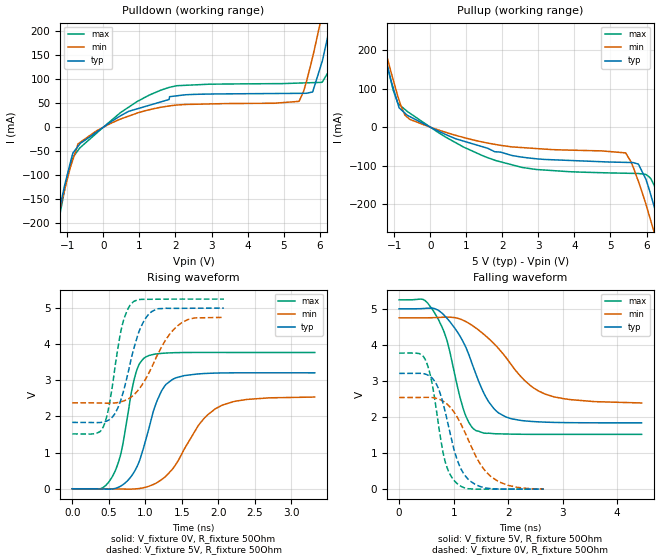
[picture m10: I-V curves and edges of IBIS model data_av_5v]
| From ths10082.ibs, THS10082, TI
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|   data_av_5v Model
[Model]   data_av_5v
Model_type   Output
Polarity   Non-Inverting
Vmeas = 2.5
Vref = 2.5
Cref = 2pF
Rref = 50
|   typ   min   max
C_comp   1.852e-12   1.852e-12   1.893e-12
[Voltage Range]   5   4.75   5.25
|Ambient Temperature   25   85   -40
|Junction Temperature
[Temperature Range]   27   125   -40
[Pullup Reference]   5   4.75   5.25
[Pulldown Reference]   0   0   0
[Power Clamp Reference]   5   4.75   5.25
[GND Clamp Reference]   0   0   0
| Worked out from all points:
|   slope of the pulldown table from 0 to 0.75 V, typ, clamps not added: 22.1 ohm
|   slope of the pullup table from 0 to 0.75 V, typ, clamps not added: 23.8 ohm
|   falling waveform, V_fixture 5V, R_fixture 50Ohm: 20-80 % time 559ps typ, 852ps min, 385ps max; typ from 5 V to 1.84 V
|   rising waveform, V_fixture 0V, R_fixture 50Ohm: 20-80 % time 298ps typ, 490ps min, 212ps max; typ from 0 V to 3.21 V
|   rising waveform, V_fixture 5V, R_fixture 50Ohm: 20-80 % time 251ps typ, 385ps min, 181ps max; typ from 1.84 V to 5 V
|   falling waveform, V_fixture 0V, R_fixture 50Ohm: 20-80 % time 339ps typ, 527ps min, 254ps max; typ from 3.21 V to 0 V
[Pulldown]
|   Voltage   I(typ)   I(min)   I(max)
-5V       -1.703A    -1.57A     -1.845A
-1.31V    -203.5mA   -203.9mA   -221.9mA
-997.5mV  -97.74mA   -106.4mA   -99.43mA
-703mV    -39.76mA   -34.62mA   -48.12mA
924mV     37.72mA    28.85mA    52.67mA
2.037V    65.07mA    45.88mA    86.03mA
5.425V    70.14mA    53.52mA    91.49mA
5.805V    72.99mA    145.8mA    92.39mA
6.053V    132.4mA    229.4mA    92.97mA
6.3V      213.6mA    313.7mA    133.8mA
6.525V    293.8mA    390.6mA    213.1mA
10V       1.666A     1.717A     1.619A
[Pullup]
|   Voltage   I(typ)   I(min)   I(max)
-5V       1.714A     1.656A     1.774A
-2.627V   730.8mA    720.8mA    765.2mA
-1.31V    203.8mA    222.1mA    205.8mA
-897.8mV  60.68mA    79.54mA    61.62mA
-703mV    36.47mA    31.19mA    46.02mA
251.7mV   -11.59mA   -8.176mA   -15.74mA
2.546V    -78.1mA    -53.24mA   -105mA
5.415V    -91.78mA   -67.03mA   -120.1mA
5.775V    -96.33mA   -141.8mA   -120.7mA
6.211V    -206.5mA   -273.6mA   -151.2mA
6.53V     -315.8mA   -375.7mA   -261.9mA
10V       -1.707A    -1.662A    -1.749A
[Ramp]
R_load = 50
|   typ   min   max
dV/dt_r   1.92515/2.95317e-10   1.52416/4.89734e-10   2.26293/2.11873e-10
dV/dt_f   1.89784/5.58635e-10   1.42308/8.5725e-10   2.23898/3.84614e-10
[Falling Waveform]
V_fixture = 5V
V_fixture_min = 4.75V
V_fixture_max = 5.25V
R_fixture = 50Ohm
|   Time   V(typ)   V(min)   V(max)
0s        5V         4.75V      5.25V
442ps     5.008V     4.75V      5.259V
642ps     5.01V      4.756V     4.908V
878ps     4.738V     4.769V     4.121V
1.2ns     4.007V     4.664V     2.121V
1.414ns   3.167V     4.46V      1.618V
1.824ns   2.113V     3.898V     1.534V
2.3ns     1.893V     3.014V     1.52V
2.676ns   1.857V     2.636V     1.518V
4.448ns   1.837V     2.389V     1.519V
[Rising Waveform]
V_fixture = 0V
V_fixture_min = 0V
V_fixture_max = 0V
R_fixture = 50Ohm
|   Time   V(typ)   V(min)   V(max)
0s        1.848nV    2.664nV    1.618nV
552ps     -4.834mV   -2.711mV   347mV
668ps     77.92mV    -6.447mV   985.8mV
868ps     536.7mV    -3.366mV   3.176V
1.01ns    1.371V     44.86mV    3.65V
1.222ns   2.701V     249.2mV    3.746V
1.422ns   3.071V     681mV      3.767V
1.732ns   3.178V     1.762V     3.773V
2.06ns    3.205V     2.317V     3.772V
3.324ns   3.208V     2.538V     3.771V
[Rising Waveform]
V_fixture = 5V
V_fixture_min = 4.75V
V_fixture_max = 5.25V
R_fixture = 50Ohm
|   Time   V(typ)   V(min)   V(max)
0s        1.837V     2.378V     1.518V
326ps     1.83V      2.376V     1.528V
428ps     1.848V     2.37V      1.728V
510ps     1.914V     2.367V     2.353V
680ps     2.547V     2.414V     4.484V
838ps     3.84V      2.588V     5.177V
938ps     4.465V     2.82V      5.24V
1.062ns   4.86V      3.252V     5.244V
1.424ns   4.993V     4.478V     5.249V
2.078ns   5V         4.743V     5.25V
[Falling Waveform]
V_fixture = 0V
V_fixture_min = 0V
V_fixture_max = 0V
R_fixture = 50Ohm
|   Time   V(typ)   V(min)   V(max)
0s        3.209V     2.54V      3.772V
360ps     3.211V     2.541V     3.761V
488ps     3.186V     2.544V     3.562V
604ps     3.08V      2.538V     2.931V
734ps     2.735V     2.493V     1.653V
838ps     2.186V     2.406V     798.3mV
1.06ns    833.5mV    2.009V     157.7mV
1.304ns   220.9mV    1.246V     6.904mV
1.688ns   10.41mV    340.8mV    397.4uV
2.652ns   431.7uV    2.134mV    162.8uV
